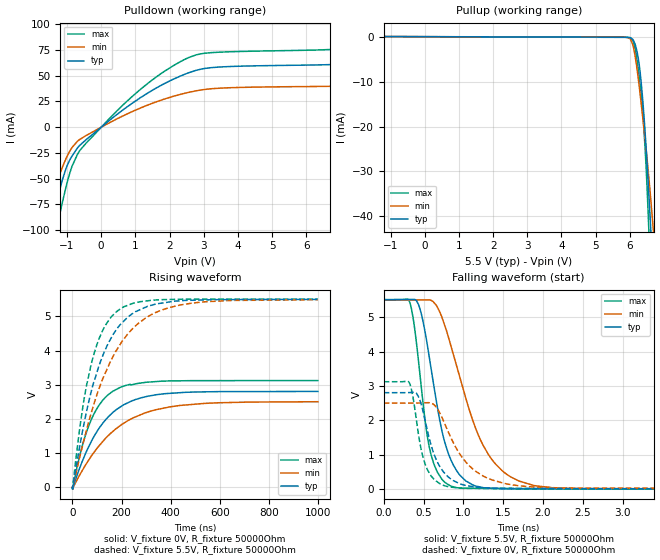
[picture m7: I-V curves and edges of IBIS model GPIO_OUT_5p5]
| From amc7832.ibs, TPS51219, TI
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|   Model
[Model]   GPIO_OUT_5p5
Model_type   Output
Polarity   Non-Inverting
Vmeas = 2.75
Vref = 5.5
Cref = 1pF
Rref = 1000000
|   typ   min   max
C_comp   1pF   1pF   1pF
[Voltage Range]   5.5   5.49   5.51
[Temperature Range]   27   125   -40
[Pullup Reference]   5.5   5.49   5.51
[Pulldown Reference]   -0   -0   -0
[Power Clamp Reference]   5.5   5.49   5.51
[GND Clamp Reference]   -0   -0   -0
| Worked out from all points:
|   slope of the pulldown table from 0 to 0.825 V, typ, clamps not added: 38.7 ohm
|   slope of the pullup table from 0 to 0.825 V, typ, clamps not added: 48 kohm
|   falling waveform, V_fixture 5.5V, R_fixture 50000Ohm: 20-80 % time 270ps typ, 475ps min, 181ps max; typ from 5.5 V to 0.008 V
|   rising waveform, V_fixture 0V, R_fixture 50000Ohm: 20-80 % time 144ns typ, 199ns min, 98.6ns max; typ from 0.004 V to 2.81 V
|   rising waveform, V_fixture 5.5V, R_fixture 50000Ohm: 20-80 % time 133ns typ, 178ns min, 93.2ns max; typ from 0.008 V to 5.5 V
|   falling waveform, V_fixture 0V, R_fixture 50000Ohm: 20-80 % time 237ps typ, 420ps min, 159ps max; typ from 2.81 V to 0.004 V
[Pulldown]
|   Voltage   I(typ)   I(min)   I(max)
-5.5V     -817.4mA   -581.8mA   -1.063A
-1.821V   -157.5mA   -108.4mA   -214.2mA
-1.655V   -129.7mA   -90.14mA   -176.9mA
-1.375V   -84.64mA   -61.01mA   -115.5mA
-1.292V   -72.27mA   -53.04mA   -98.94mA
-913mV    -31.49mA   -23.01mA   -43.96mA
-632.5mV  -17.82mA   -12.06mA   -22.96mA
1.166V    28.92mA    18.78mA    37.11mA
2.783V    55.15mA    35.25mA    70.14mA
8.129V    64.39mA    41.7mA     80.74mA
10.03V    84.1mA     53.55mA    108.1mA
10.98V    102.5mA    65.77mA    133.6mA
[Pullup]
|   Voltage   I(typ)   I(min)   I(max)
-5.5V     114.6uA    1.467mA    144uA
-4.724V   98.35uA    93.42uA    123.7uA
6.017V    -226.8uA   -554.6uA   -268.7uA
6.149V    -1.572mA   -4.05mA    -2.456mA
6.298V    -7.658mA   -12.53mA   -10.54mA
6.413V    -17.59mA   -20.43mA   -20.66mA
6.463V    -23.1mA    -23.99mA   -27.02mA
6.529V    -31.34mA   -29.1mA    -37.78mA
6.578V    -37.99mA   -33.2mA    -47.05mA
6.611V    -42.58mA   -36.04mA   -53.56mA
6.71V     -56.99mA   -44.99mA   -74.09mA
10.98V    -814.2mA   -580.8mA   -1.057A
[Ramp]
R_load = 50000
|   typ   min   max
dV/dt_r   1.68108/1.44268e-07   1.49995/1.98785e-07   1.8721/9.85891e-08
dV/dt_f   3.29527/2.69254e-10   3.28758/4.73328e-10   3.30186/1.8092e-10
[Falling Waveform]
V_fixture = 5.5V
V_fixture_min = 5.49V
V_fixture_max = 5.51V
R_fixture = 50000Ohm
C_fixture = 0F
|   Time   V(typ)   V(min)   V(max)
0s        5.5V       5.49V      5.51V
327.2ps   5.511V     5.497V     5.43V
444.6ps   5.316V     5.499V     3.559V
561.2ps   3.997V     5.501V     1.358V
727.1ps   1.743V     5.02V      302.3mV
960.8ps   399mV      3.215V     33.48mV
1.319ns   33.85mV    994.4mV    27.18mV
1.608ns   15.61mV    343.1mV    22.11mV
2.008ns   15.61mV    74.53mV    15.07mV
1us       7.874mV    10.86mV    6.893mV
[Rising Waveform]
V_fixture = 0V
V_fixture_min = 0V
V_fixture_max = 0V
R_fixture = 50000Ohm
C_fixture = 0F
|   Time   V(typ)   V(min)   V(max)
0s        3.959mV    4.903mV    3.844mV
573.5ps   -26.62mV   3.379mV    -54.53mV
1.075ns   -42.71mV   -54.44mV   -32.45mV
40.2ns    761.5mV    491.4mV    1.215V
81.06ns   1.402V     956.7mV    2.049V
133.5ns   1.962V     1.421V     2.628V
194.4ns   2.348V     1.804V     2.924V
296.7ns   2.648V     2.18V      3.071V
438.5ns   2.77V      2.396V     3.117V
1us       2.806V     2.505V     3.124V
[Rising Waveform]
V_fixture = 5.5V
V_fixture_min = 5.49V
V_fixture_max = 5.51V
R_fixture = 50000Ohm
C_fixture = 0F
|   Time   V(typ)   V(min)   V(max)
0s        7.874mV    10.86mV    6.893mV
26.38ns   1.066V     778.4mV    1.544V
45.21ns   1.788V     1.332V     2.483V
81.06ns   2.927V     2.282V     3.729V
123.7ns   3.856V     3.182V     4.601V
182.3ns   4.649V     4.045V     5.157V
267.4ns   5.174V     4.792V     5.42V
395.3ns   5.425V     5.262V     5.498V
540.6ns   5.485V     5.431V     5.507V
1us       5.5V       5.49V      5.51V
[Falling Waveform]
|Gnd
V_fixture = 0V
V_fixture_min = 0V
V_fixture_max = 0V
R_fixture = 50000Ohm
C_fixture = 0F
|   Time   V(typ)   V(min)   V(max)
0s        2.806V     2.505V     3.124V
320.9ps   2.809V     2.505V     3.096V
411.1ps   2.791V     2.505V     2.007V
508.2ps   2.113V     2.511V     815.6mV
601.9ps   1.228V     2.496V     369.2mV
699.5ps   680.7mV    2.238V     170.2mV
967.1ps   152.1mV    983.8mV    34.72mV
1.248ns   46.76mV    386.9mV    23.99mV
2.435ns   19.97mV    35.21mV    9.267mV
1us       3.959mV    4.903mV    3.844mV
